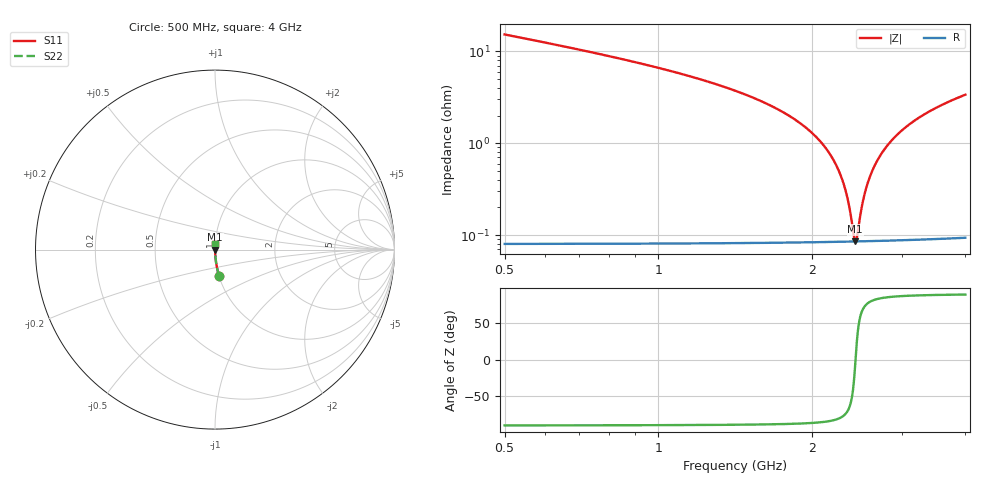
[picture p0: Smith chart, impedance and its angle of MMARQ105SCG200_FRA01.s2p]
! MMARQ105SCG200_FRA01  S-PARAMETER MODEL  ( General Type )
! Model Generated by TAIYO YUDEN Corporation (http://www.ty-top.com)
! Version 1.0
! TAIYO YUDEN Control No. 200326
! Copyright(c) 2020 TAIYO YUDEN CO.,LTD. All Rights Reserved.
! Product Description (link to TY-COMPAS)
! https://ds.yuden.co.jp/TYCOMPAS/or/detail?pn=MMARQ105SCG200JFRA01&u=M
! Products Name : Multilayer Ceramic Capacitors
! Characteristics :
!  Capacitance : 20 pF , Rated Voltage : 250V , TCC : CG / C0G
!  Case Size : 1.0 x 0.5 / 0.039 x 0.02 [mm/inch] , Thickness : 0.5 / 0.02 [mm/inch]
!  (Conditions: Temperature = 25 degC , DC Bias Current/Voltage = 0A / 0V)
! External Node Assignments :
!  1  o---| |---o  2
! GND o---------o GND
! Frequency Range : 500MHz  -  4GHz  [ 401 STEP ]
# MHz S RI R 50
! Freq[MHz].  S11 Real  S11 Imag  S21 Real  S21 Imag  S12 Real  S12 Imag  S22 Real  S22 Imag
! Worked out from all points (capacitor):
!   401 points, 500 MHz to 4 GHz, reference 50 ohm
!   read as one part in series: C = 20 pF near 517.5 MHz
!   lowest |Z| = 85.7 mohm at 2.434 GHz (marker M1)
!   series resonance near 2.437 GHz, so ESL is about 210 pH
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500  0.0235 -0.1489  0.9765 0.1489  0.9765 0.1489  0.0235 -0.1489
753.75  0.00983 -0.0945  0.9902 0.0945  0.9902 0.0945  0.00983 -0.0945
1086.25  0.00424 -0.0585  0.9958 0.0585  0.9958 0.0585  0.00424 -0.0585
1672.5  0.00146 -0.0251  0.9985 0.0251  0.9985 0.0251  0.00146 -0.0251
1873.75  0.00113 -0.0173  0.9989 0.0173  0.9989 0.0173  0.00113 -0.0173
2031.25  0.00098 -0.0119  0.999 0.0119  0.999 0.0119  0.00098 -0.0119
2153.75  0.000907 -0.00807  0.9991 0.00807  0.9991 0.00807  0.000907 -0.00807
2250  0.000873 -0.0052  0.9991 0.0052  0.9991 0.0052  0.000873 -0.0052
2293.75  0.000863 -0.00394  0.9991 0.00394  0.9991 0.00394  0.000863 -0.00394
2337.5  0.000856 -0.00271  0.9991 0.00271  0.9991 0.00271  0.000856 -0.00271
2372.5  0.000853 -0.00174  0.9991 0.00174  0.9991 0.00174  0.000853 -0.00174
2416.25  0.000852 -0.000545  0.9991 0.000545  0.9991 0.000545  0.000852 -0.000545
2433.75  0.000853 -7.41e-05  0.9991 7.41e-05  0.9991 7.41e-05  0.000853 -7.41e-05
2451.25  0.000854 0.000393  0.9991 -0.000393  0.9991 -0.000393  0.000854 0.000393
2503.75  0.000859 0.00178  0.9991 -0.00178  0.9991 -0.00178  0.000859 0.00178
2530  0.000863 0.00246  0.9991 -0.00246  0.9991 -0.00246  0.000863 0.00246
2591.25  0.000876 0.00402  0.9991 -0.00402  0.9991 -0.00402  0.000876 0.00402
2696.25  0.000908 0.00662  0.9991 -0.00662  0.9991 -0.00662  0.000908 0.00662
2836.25  0.00097 0.00995  0.999 -0.00995  0.999 -0.00995  0.00097 0.00995
3081.25  0.00112 0.0155  0.9989 -0.0155  0.9989 -0.0155  0.00112 0.0155
3422.5  0.00141 0.0226  0.9986 -0.0226  0.9986 -0.0226  0.00141 0.0226
4000  0.00207 0.0336  0.9979 -0.0336  0.9979 -0.0336  0.00207 0.0336
